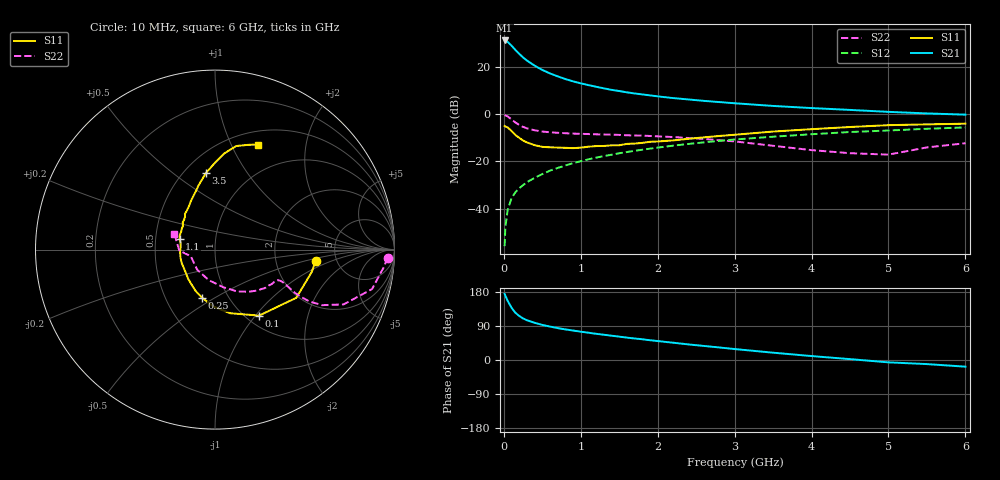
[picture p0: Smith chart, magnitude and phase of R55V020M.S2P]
! SIEMENS Small Signal Semiconductors
! BFR183
! Si NPN RF Bipolar Junction Transistor in SOT23
! VCE = 5 V  IC = 20 mA
! Common Emitter S-Parameters:  May  1996
# GHz  S  MA  R  50
!  f  S11  S21  S12  S22
! GHz  MAG  ANG  MAG  ANG  MAG  ANG  MAG  ANG
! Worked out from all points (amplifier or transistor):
!   36 points, 10 MHz to 6 GHz, reference 50 ohm
!   highest |S21| = 31.3 dB at 10 MHz (marker M1)
!   |S21| within 3 dB of that: start of sweep to 122.1 MHz
!   unconditionally stable (mu >= 1): 608.1 MHz to 2.437 GHz
!   at 250 MHz: K = 0.80, MSG = 27.1 dB, |S12| = -30.1 dB
!   at 1.4 GHz: K = 1.04, MAG = 12.5 dB, |S12| = -17.1 dB
!   at 6 GHz: K = 0.90, MSG = 2.7 dB, |S12| = -5.6 dB
!   S11 on the Smith chart (normalised r, x): 10 MHz: 3.46, -0.64; 100 MHz: 1.14, -1.04; 250 MHz: 0.76, -0.44; 1.1 GHz: 0.67, +0.08; 3.5 GHz: 0.63, +0.67; 6 GHz: 0.65, +1.27
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0.01  0.564 -6.4  36.81 174.6  0.0016 88.0  0.9631 -2.7
0.02  0.5538 -12.8  36.59 169.5  0.0041 87.3  0.9458 -5.9
0.05  0.5264 -30.7  34.31 156.0  0.0094 77.9  0.9023 -14.1
0.1  0.442 -56.3  28.57 138.0  0.0167 71.8  0.7785 -23.1
0.15  0.3644 -76.6  23.19 124.7  0.0222 68.4  0.6705 -27.5
0.2  0.3176 -91.5  19.16 116.2  0.0272 68.6  0.5952 -28.8
0.25  0.2785 -104.7  16.06 109.7  0.0314 68.3  0.5412 -28.8
0.3  0.2539 -115.4  13.83 104.9  0.0363 69.4  0.5046 -28.4
0.4  0.2217 -132.2  10.75 98.2  0.045 70.2  0.4585 -27.0
0.5  0.2039 -145.8  8.712 92.6  0.0541 71.1  0.4312 -26.0
0.6  0.2001 -159.0  7.363 88.2  0.0639 71.3  0.4164 -25.6
0.7  0.1969 -168.7  6.373 84.2  0.0729 71.3  0.4055 -25.5
0.8  0.1947 -177.1  5.597 80.7  0.0823 70.7  0.397 -25.7
0.9  0.1917 176.0  4.996 77.7  0.0922 70.3  0.39 -25.9
1.1  0.2058 163.2  4.16 72.0  0.1111 69.3  0.3813 -27.9
1.3  0.213 152.2  3.547 66.6  0.1301 67.6  0.373 -29.7
1.6  0.2359 139.6  2.922 59.1  0.1586 64.9  0.3593 -33.8
2.2  0.2792 121.7  2.21 45.6  0.2163 58.8  0.3298 -43.6
3.5  0.431 96.6  1.505 19.3  0.3349 42.6  0.2151 -77.4
4.5  0.5383 84.5  1.239 2.3  0.4215 30.0  0.1498 -131.6
5.5  0.6119 72.5  1.044 -10.8  0.4935 18.4  0.1988 -178.4
6  0.6328 67.7  0.984 -17.6  0.5276 11.0  0.2437 158.5
